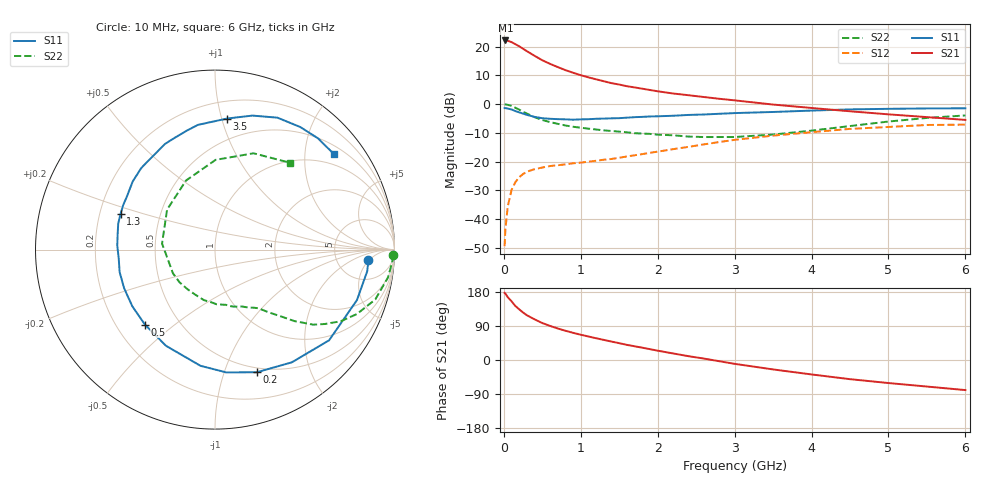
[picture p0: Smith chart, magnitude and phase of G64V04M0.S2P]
! SIEMENS Small Signal Semiconductors
! BFG193
! Si NPN RF Bipolar Junction Transistor in SOT223
! VCE = 4 V  IC = 4 mA
! Common Emitter S-Parameters:  August  1996
# GHz  S  MA  R  50
!  f  S11  S21  S12  S22
! GHz  MAG  ANG  MAG  ANG  MAG  ANG  MAG  ANG
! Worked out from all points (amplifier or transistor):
!   36 points, 10 MHz to 6 GHz, reference 50 ohm
!   highest |S21| = 22.2 dB at 20 MHz (marker M1)
!   |S21| within 3 dB of that: start of sweep to 256.6 MHz
!   unconditionally stable (mu >= 1): 1.199 GHz to 2.527 GHz
!   at 250 MHz: K = 0.29, MSG = 21.8 dB, |S12| = -24.3 dB
!   at 1.4 GHz: K = 1.09, MAG = 11.4 dB, |S12| = -19.0 dB
!   at 6 GHz: K = 0.89, MSG = 0.8 dB, |S12| = -7.1 dB
!   S11 on the Smith chart (normalised r, x): 10 MHz: 11, -5; 200 MHz: 0.45, -1.30; 500 MHz: 0.32, -0.40; 1.3 GHz: 0.29, +0.17; 3.5 GHz: 0.33, +1.04; 6 GHz: 0.70, +2.69
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0.01  0.8571 -4.0  12.85 177.0  0.0034 90.8  0.9924 -1.8
0.02  0.8566 -8.1  12.86 175.2  0.0066 84.1  0.9908 -3.6
0.05  0.8394 -19.6  12.71 166.0  0.0165 78.6  0.9766 -9.1
0.1  0.812 -38.5  12.03 154.9  0.0322 71.0  0.9352 -17.3
0.15  0.7601 -55.7  11.07 142.5  0.0442 61.6  0.8685 -24.4
0.2  0.7221 -71.1  10.17 133.7  0.0537 55.9  0.8061 -29.7
0.25  0.6873 -84.7  9.219 125.2  0.0612 50.2  0.7394 -34.1
0.3  0.6525 -97.1  8.361 118.1  0.0671 46.0  0.6885 -37.4
0.4  0.6017 -116.9  6.943 107.2  0.0743 40.8  0.5953 -42.0
0.5  0.572 -133.0  5.816 97.5  0.0793 36.9  0.5317 -44.9
0.6  0.5585 -145.6  5.042 90.0  0.0841 35.2  0.4892 -47.4
0.7  0.5503 -156.9  4.432 83.2  0.0868 34.2  0.4564 -49.7
0.9  0.5386 -174.9  3.527 71.7  0.0939 33.7  0.4058 -53.6
1.1  0.5487 171.4  2.934 62.0  0.1002 34.6  0.3759 -59.2
1.3  0.5626 159.2  2.511 53.0  0.1084 35.4  0.351 -64.5
1.6  0.5838 144.1  2.058 39.9  0.1235 36.0  0.3252 -75.4
2.2  0.6303 121.5  1.537 17.3  0.1654 33.7  0.2883 -102.3
3  0.7014 97.8  1.168 -10.1  0.24 23.1  0.2689 -150.7
3.5  0.7334 84.7  0.987 -24.9  0.2848 11.7  0.2969 173.5
4.5  0.8131 64.7  0.754 -50.6  0.3726 -9.6  0.4173 112.8
5.5  0.8448 47.2  0.597 -70.1  0.4357 -36.3  0.5779 68.2
6  0.8498 38.7  0.534 -79.4  0.4414 -51.3  0.6388 49.3
